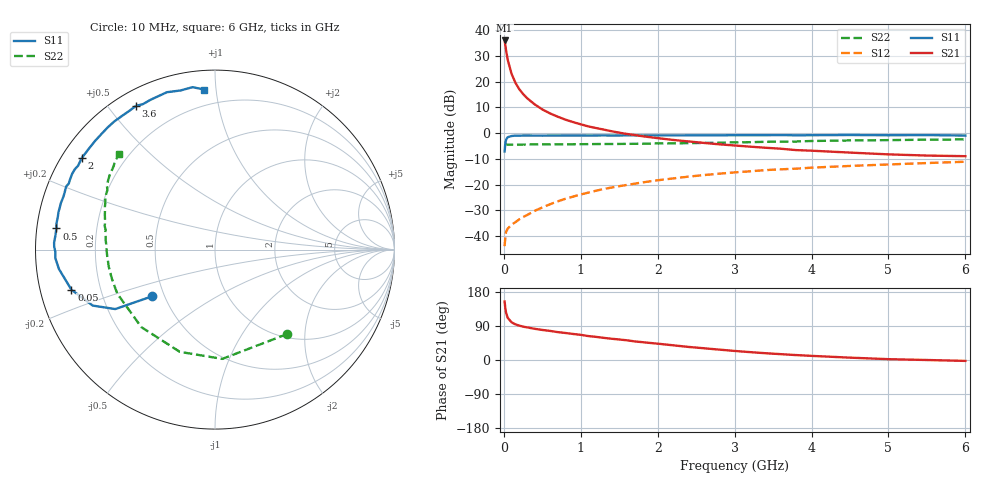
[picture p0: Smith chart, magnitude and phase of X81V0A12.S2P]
! SIEMENS Small Signal Semiconductors
! BFP136W
! Si NPN RF Bipolar Junction Transistor in SOT343
! VCE = 1 V  IC = 120 mA
! Common Emitter S-Parameters:  September  1994
# GHz  S  MA  R  50
!  f  S11  S21  S12  S22
! GHz  MAG  ANG  MAG  ANG  MAG  ANG  MAG  ANG
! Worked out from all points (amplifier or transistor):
!   40 points, 10 MHz to 6 GHz, reference 50 ohm
!   highest |S21| = 35.9 dB at 10 MHz (marker M1)
!   |S21| within 3 dB of that: start of sweep to 25.01 MHz
!   unconditionally stable (mu >= 1): 361.3 MHz to 4.368 GHz; 4.61 GHz to end of sweep
!   at 200 MHz: K = 0.80, MSG = 25.3 dB, |S12| = -33.5 dB
!   at 1.5 GHz: K = 1.16, MAG = 8.0 dB, |S12| = -20.6 dB
!   at 6 GHz: K = 1.06, MAG = -0.4 dB, |S12| = -11.1 dB
!   S11 on the Smith chart (normalised r, x): 10 MHz: 0.43, -0.28; 50 MHz: 0.09, -0.14; 500 MHz: 0.06, +0.07; 2 GHz: 0.06, +0.31; 3.6 GHz: 0.06, +0.59; 6 GHz: 0.10, +0.93
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0.01  0.4388 -143.5  62.52 154.4  0.0064 60.7  0.6192 -49.4
0.02  0.6471 -149.2  49.77 135.6  0.0098 48.1  0.6103 -86.2
0.03  0.7492 -155.4  39.37 123.9  0.0122 42.1  0.6024 -109.0
0.05  0.8307 -164.4  26.53 111.4  0.014 33.6  0.5958 -133.5
0.1  0.8761 -172.9  14.12 99.5  0.0166 35.0  0.5971 -155.7
0.15  0.8907 -176.9  9.503 94.1  0.0187 40.4  0.5969 -164.0
0.2  0.8894 -179.1  7.109 90.7  0.0212 43.8  0.5981 -168.4
0.25  0.8962 178.9  5.729 88.1  0.0234 47.2  0.6 -171.3
0.3  0.8973 177.5  4.786 86.2  0.0256 50.7  0.5995 -173.2
0.4  0.8922 174.7  3.608 82.4  0.0309 54.9  0.6014 -175.9
0.5  0.8918 172.4  2.875 79.3  0.0361 58.2  0.6025 -177.9
0.7  0.8945 168.1  2.077 73.6  0.0472 61.4  0.6046 179.6
0.9  0.8961 164.9  1.632 68.7  0.0585 62.4  0.6067 177.3
1.1  0.8945 160.7  1.345 63.1  0.0702 62.3  0.61 175.6
1.5  0.8973 154.2  1.017 54.1  0.0932 60.9  0.615 172.2
2  0.9007 145.3  0.797 43.1  0.1215 56.7  0.6288 167.8
2.2  0.8999 141.9  0.736 38.8  0.1319 54.8  0.6304 166.1
3.2  0.9073 124.9  0.545 20.8  0.1812 44.3  0.6654 156.6
3.6  0.9137 118.8  0.497 15.4  0.1981 40.2  0.681 152.9
4.5  0.9169 107.0  0.418 6.2  0.2304 31.3  0.7187 144.8
5.5  0.9136 97.9  0.366 0.0  0.2621 23.2  0.7441 138.2
6  0.8939 93.8  0.356 -2.4  0.278 18.8  0.7534 135.3
